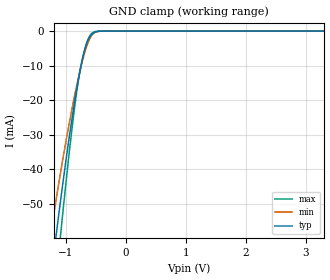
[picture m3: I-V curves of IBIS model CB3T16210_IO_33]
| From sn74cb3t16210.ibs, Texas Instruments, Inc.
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[Model]   CB3T16210_IO_33
Model_type  Terminator
| variable   typ   min   max
C_comp   3.72pF   3.03pF   4.47pF
| C_tri-state   3.72pF   3.03pF   4.47pF
[Temperature Range]   40   100   -40
| Ambient temperature   25   85   -40
[Voltage range]   3.3   3   3.6
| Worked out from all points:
|   GND clamp passes 1 mA (typ) near -0.57 V on its own axis
[GND Clamp]
| CB3T16210_IO_33
|   Voltage   I(typ)   I(min)   I(max)
-5.5V     -844.5mA   -703.3mA   -992.6mA
-1.245V   -70.99mA   -57.97mA   -87.24mA
-1.15V    -57.58mA   -47.56mA   -70.02mA
-1.08V    -48.11mA   -40.21mA   -57.77mA
-910mV    -26.86mA   -23.7mA    -30.18mA
-800mV    -14.95mA   -14.32mA   -15.38mA
-740mV    -9.421mA   -9.824mA   -9.498mA
-680mV    -5.043mA   -5.952mA   -5.039mA
-620mV    -2.246mA   -2.942mA   -2.024mA
-565mV    -887.1uA   -1.181mA   -624.9uA
-395mV    -15.06uA   -22.69uA   -2.774uA
3.3V      247pA      10.93nA    95.08pA
